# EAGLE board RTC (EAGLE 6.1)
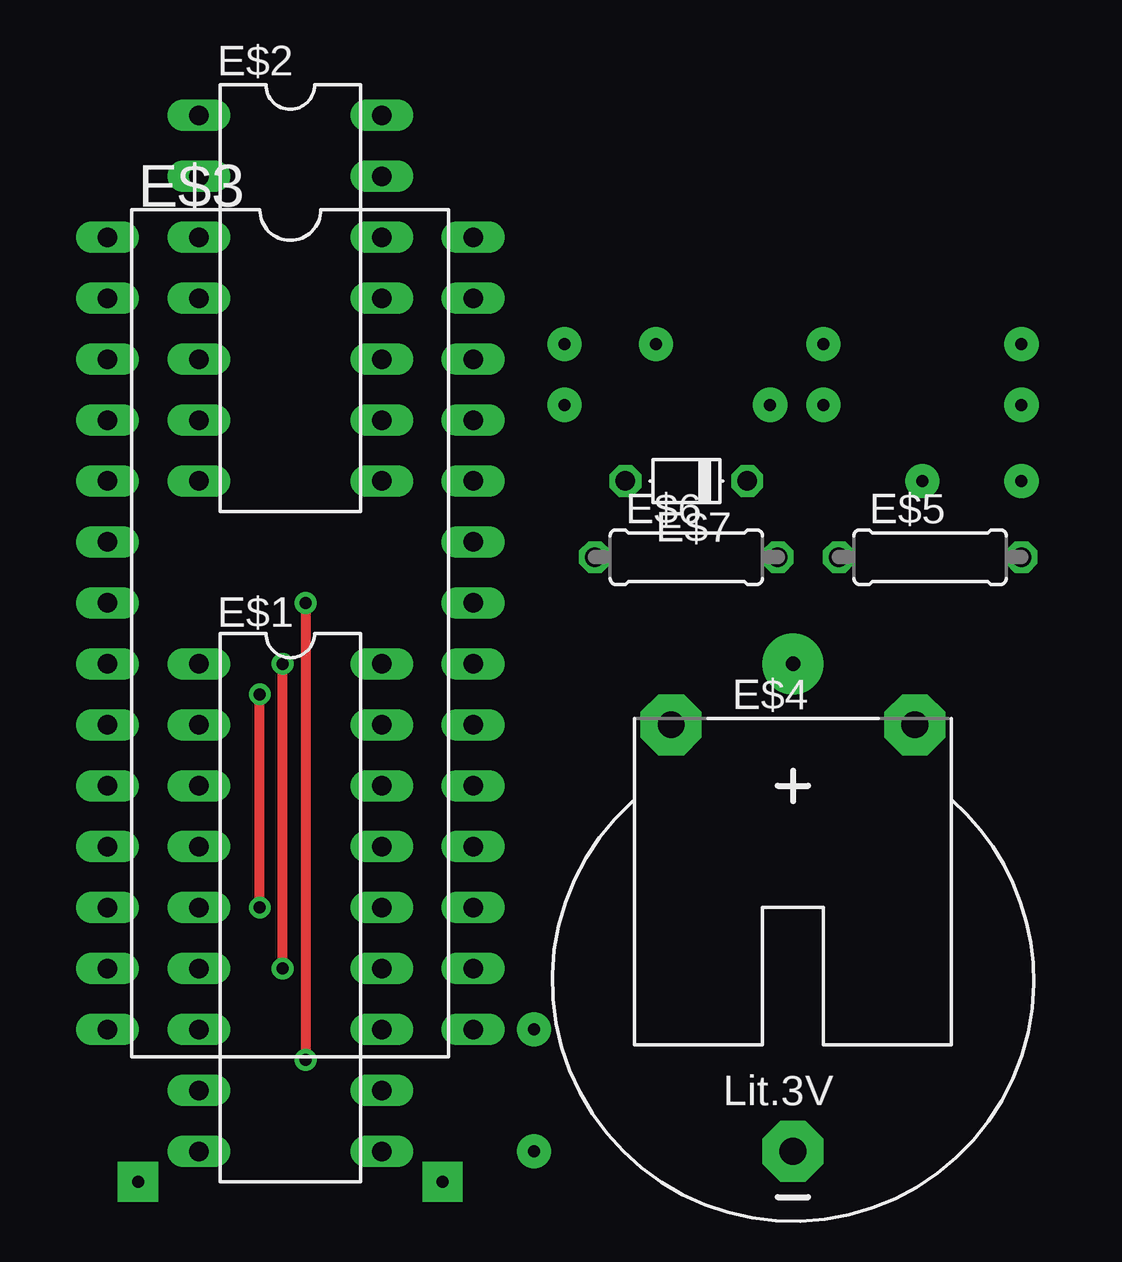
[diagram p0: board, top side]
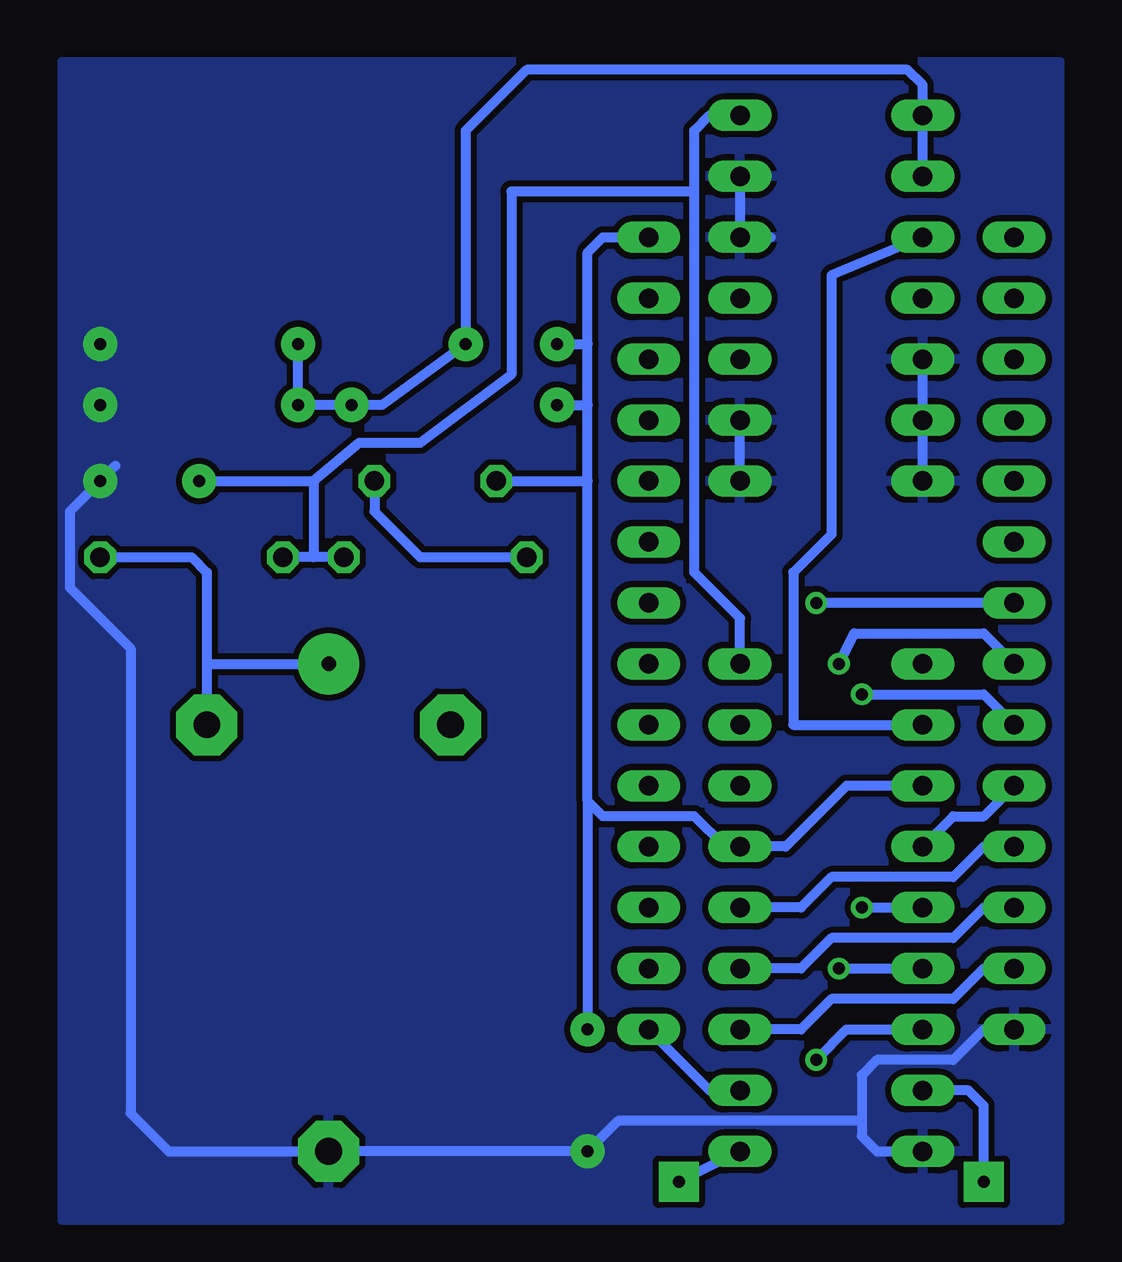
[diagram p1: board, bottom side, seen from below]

No outline drawn. Coordinates in mm, seen from the top.
Copper layers (1*16): Top 0.035mm / dielectric 1.5mm / Bottom 0.035mm
Design rules: minimum track width 10mil, minimum drill 24mil, track to track 8mil, track to pad 8mil, pad to pad 8mil, via to via 8mil, smd to smd 8mil, copper to edge 40mil, drill to drill 8mil, minimum pad ring 10mil, minimum via ring 8mil, stop-mask expansion 4mil, vias tented up to drill 0mil, thermal gap 10mil

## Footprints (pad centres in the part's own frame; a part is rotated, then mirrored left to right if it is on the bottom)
DIL18 = drill 0.813 long: 1 -10.16,-3.81; 2 -7.62,-3.81; 3 -5.08,-3.81; 4 -2.54,-3.81; 5 0,-3.81; 6 2.54,-3.81; 7 5.08,-3.81; 8 7.62,-3.81; 9 10.16,-3.81; 10 10.16,3.81; 11 7.62,3.81; 12 5.08,3.81; 13 2.54,3.81; 14 0,3.81; 15 -2.54,3.81; 16 -5.08,3.81; 17 -7.62,3.81; 18 -10.16,3.81
DIL14 = drill 0.813 long: 1 -7.62,-3.81; 2 -5.08,-3.81; 3 -2.54,-3.81; 4 0,-3.81; 5 2.54,-3.81; 6 5.08,-3.81; 7 7.62,-3.81; 8 7.62,3.81; 9 5.08,3.81; 10 2.54,3.81; 11 0,3.81; 12 -2.54,3.81; 13 -5.08,3.81; 14 -7.62,3.81
DIL28-6 = drill 0.813 long: 1 -16.51,-7.62; 2 -13.97,-7.62; 3 -11.43,-7.62; 4 -8.89,-7.62; 5 -6.35,-7.62; 6 -3.81,-7.62; 7 -1.27,-7.62; 8 1.27,-7.62; 9 3.81,-7.62; 10 6.35,-7.62; 11 8.89,-7.62; 12 11.43,-7.62; 13 13.97,-7.62; 14 16.51,-7.62; 15 16.51,7.62; 16 13.97,7.62; 17 11.43,7.62; 18 8.89,7.62; 19 6.35,7.62; 20 3.81,7.62; 21 1.27,7.62; 22 -1.27,7.62; 23 -3.81,7.62; 24 -6.35,7.62; 25 -8.89,7.62; 26 -11.43,7.62; 27 -13.97,7.62; 28 -16.51,7.62
CR2032H = drill 1.118 pad 2.54 octagon: + 5.08,10.795; +@1 -5.08,10.795; - 0,-6.985
0207/7 = drill 0.813 octagon: 1 -3.81,0; 2 3.81,0
D-5 = drill 0.813 octagon: A 2.54,0; C -2.54,0

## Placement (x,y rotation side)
E$1  [DIL18]  53.34,33.02 270 top
E$2  [DIL14]  53.34,58.42 270 top
E$3  [DIL28-6]  53.34,44.45 270 top
E$4  [CR2032H]  74.3,29.84 0 top
E$5  [0207/7]  80.01,47.62 0 top
E$6  [0207/7]  69.85,47.62 0 top
E$7  [D-5]  69.85,50.8 180 top

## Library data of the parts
E$1-E$3 = 74xx-us
E$4 = battery
E$5 E$6 = rcl
E$7 = diode

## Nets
GND: E$1.9 E$2.5 E$2.7 E$2.8 E$2.9 E$2.12 E$2.13 E$3.14 E$4.-
S$1: E$1.4 E$3.10
S$2: E$1.5 E$3.9
S$6: E$1.7 E$3.7
S$7: E$1.14 E$3.11
S$8: E$1.13 E$3.12
S$9: E$1.12 E$3.13
S$10: E$1.11 E$3.15
S$11: E$6.1 E$7.C
S$12: E$1.3 E$1.15 E$3.28 E$7.A
S$13: E$1.6 E$3.8
S$15: E$1.18 E$2.14 E$5.1 E$6.2
S$18: E$1.8
S$19: E$1.10
S$20: E$1.2 E$2.3
S$25: E$4.+ E$5.2
S$26: E$2.1 E$2.2

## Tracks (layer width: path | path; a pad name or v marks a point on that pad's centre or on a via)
GND  (via drill 0.5 pad 1.42)
  Bottom 0.406: E$3.14 46.99,27.94 48.26,26.67 51.44,26.67 52.07,26.04 52.07,24.13 | 52.07,24.13 52.07,23.5 51.44,22.86 E$1.9 | 52.07,24.13 62.23,24.13 v63.5,22.86 E$4.- 80.96,22.86 82.55,24.45 82.55,43.81 85.09,46.35 85.09,49.53 v83.82,50.8 83.19,51.44 | E$2.7 E$2.5 | E$2.13 E$2.12 55.88,60.96 | E$2.8 E$2.9
  other vias: 83.82,56.52 83.82,53.98
  pour Bottom (isolate 0.254): 43.81,68.26 85.41,68.26 85.41,20 43.81,20
S$1
  Bottom 0.406: E$1.4 48.26,36.83 46.99,36.83 E$3.10
S$2  (via drill 0.5 pad 0.7)
  Top 0.406: v52.07,33.02 v52.07,41.91
  Bottom 0.406: v52.07,41.91 46.99,41.91 E$3.9 | v52.07,33.02 E$1.5
S$6  (via drill 0.5 pad 0.7)
  Top 0.406: v53.98,45.72 v53.98,26.67
  Bottom 0.406: v53.98,26.67 52.7,27.94 E$1.7 | E$3.7 v53.98,45.72
S$7
  Bottom 0.406: E$3.11 46.99,35.56 48.26,34.29 53.34,34.29 54.61,33.02 E$1.14
S$8
  Bottom 0.406: E$3.12 46.99,33.02 48.26,31.75 53.34,31.75 54.61,30.48 E$1.13
S$9
  Bottom 0.406: E$3.13 46.99,30.48 48.26,29.21 53.34,29.21 54.61,27.94 E$1.12
S$10
  Bottom 0.406: E$1.11 58.42,25.4 E$3.15
S$11
  Bottom 0.406: E$7.C 72.39,49.53 70.48,47.62 E$6.1
S$12  (via drill 0.5 pad 1.42)
  Bottom 0.406: E$1.3 52.7,38.1 55.24,35.56 E$1.15 57.78,35.56 59.05,36.83 62.87,36.83 63.5,37.47 | 63.5,37.47 63.5,50.8 | 63.5,50.8 63.5,53.98 | 63.5,53.98 63.5,56.52 | 63.5,56.52 63.5,60.33 62.87,60.96 E$3.28 | 63.5,37.47 v63.5,27.94 | E$7.A 63.5,50.8 | v64.77,56.52 63.5,56.52 | v64.77,53.98 63.5,53.98
S$13  (via drill 0.5 pad 0.7)
  Top 0.406: v53.02,30.48 v53.02,43.18
  Bottom 0.406: v53.02,43.18 52.39,44.45 46.99,44.45 E$3.8 | v53.02,30.48 E$1.6
S$15  (via drill 0.5 pad 1.42)
  Bottom 0.406: E$1.18 57.15,45.09 59.05,46.99 59.05,62.87 | 59.05,62.87 59.05,65.41 58.42,66.04 E$2.14 | 59.05,62.87 66.67,62.87 66.67,55.24 70.48,52.39 73.03,52.39 74.93,50.8 | E$6.2 74.93,47.62 | 74.93,47.62 E$5.1 | 74.93,50.8 74.93,47.62 | v79.69,50.8 74.93,50.8
S$18  (via drill 0.5 pad 1.68)
  Bottom 0.406: v46.99,21.59 46.99,24.77 47.62,25.4 E$1.8
S$19  (via drill 0.5 pad 1.68)
  Bottom 0.406: E$1.10 v59.69,21.59
S$20
  Bottom 0.406: E$2.3 53.34,59.37 53.34,48.58 54.93,46.99 54.93,40.64 E$1.2
S$25  (via drill 0.6 pad 2.54)
  Bottom 0.406: E$5.2 80.01,47.62 79.38,46.99 79.38,43.18 | 79.38,43.18 E$4.+ | 79.38,43.18 v74.3,43.18
S$26  (via drill 0.5 pad 1.42)
  Bottom 0.406: E$2.2 E$2.1 49.53,67.31 50.16,67.94 66.04,67.94 68.58,65.41 v68.58,56.52 72.07,53.98 v73.34,53.98 v75.56,53.98 v75.56,56.52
